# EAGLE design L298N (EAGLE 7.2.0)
CNAME: L298 STEPPER MOTOR BOARD; CREVISION: 1.0; DESIGNER: RODNEYD
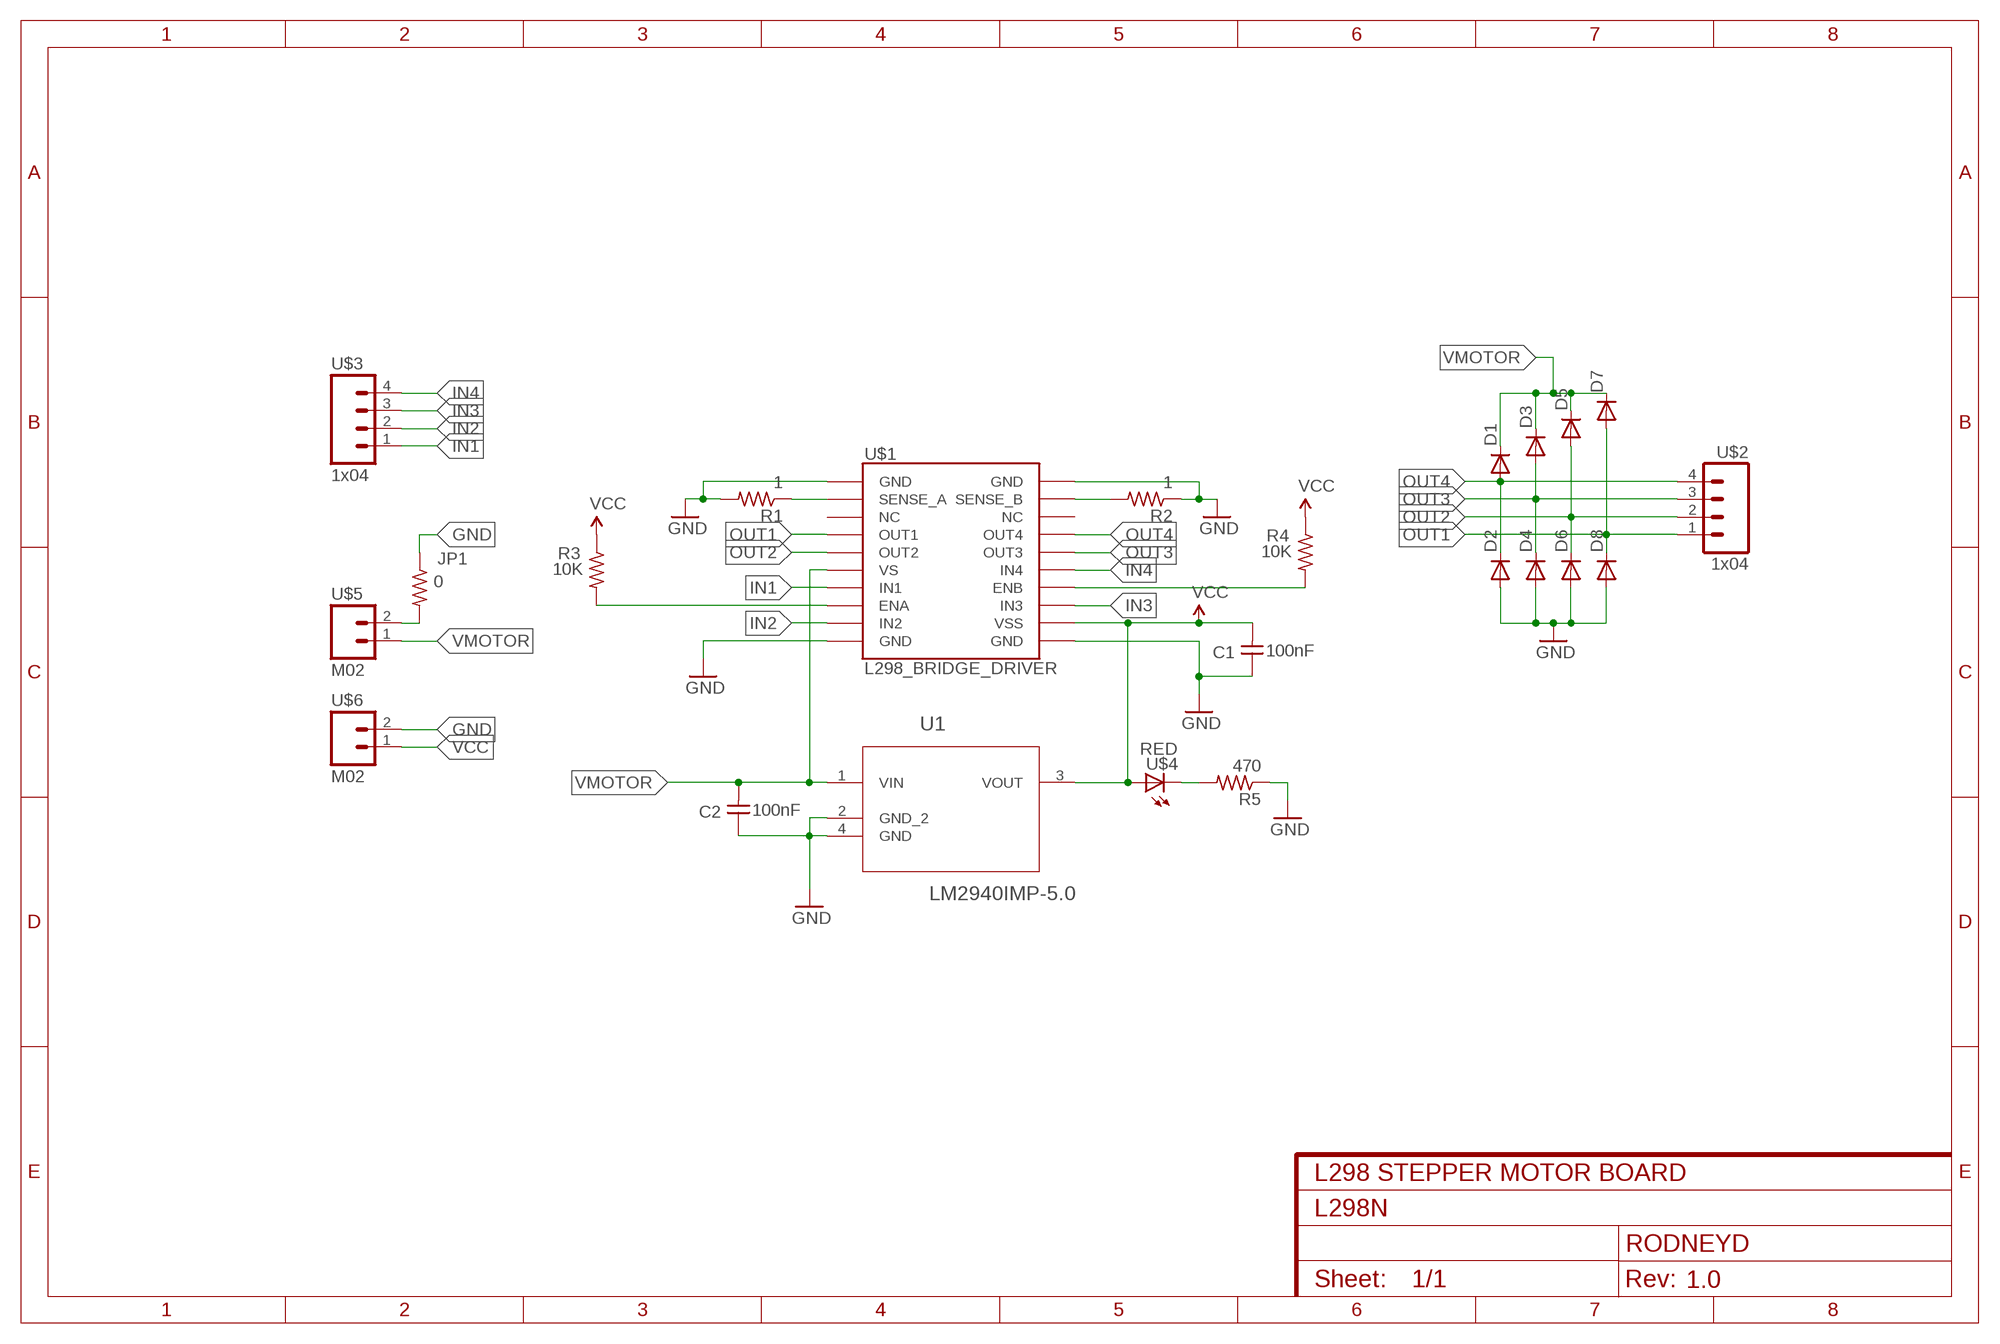
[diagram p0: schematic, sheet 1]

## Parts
C1  100nF  CAPFAB  [C1206FAB]
C2  100nF  CAPFAB  [C1206FAB]
D1  DIODESOD123  [SOD123]
D2  DIODESOD123  [SOD123]
D3  DIODESOD123  [SOD123]
D4  DIODESOD123  [SOD123]
D5  DIODESOD123  [SOD123]
D6  DIODESOD123  [SOD123]
D7  DIODESOD123  [SOD123]
D8  DIODESOD123  [SOD123]
JP1  0  RESISTOR1206FAB  [R1206FAB]
R1  1  RESISTOR1206FAB  [R1206FAB]
R2  1  RESISTOR1206FAB  [R1206FAB]
R3  10K  RESISTOR1206FAB  [R1206FAB]
R4  10K  RESISTOR1206FAB  [R1206FAB]
R5  470  RESISTOR1206FAB  [R1206FAB]
U1  LM2940IMP-5.0  [SOT230P696X180-4N]
U$1  L298_BRIDGE_DRIVER  [POWERSO20]
U$2  1x04  M041X04_SMD_STRAIGHT_ALT  [1X04_SMD_STRAIGHT_ALT]
U$3  1x04  M041X04_SMD_STRAIGHT_ALT  [1X04_SMD_STRAIGHT_ALT]
U$4  RED  LED  [LED1206]
U$5  M02  [1X02_SMD_FLAT_PADS]
U$6  M02  [1X02_SMD_FLAT_PADS]

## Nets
GND: C1.1 C2.1 D2.ANODE(A) D4.ANODE(A) D6.ANODE(A) D8.ANODE(A) JP1.1 R1.2 R2.1 R5.1 U1.2(GND_2) U1.4(GND) U$1.1(GND) U$1.10(GND) U$1.11(GND) U$1.20(GND) U$6.2
IN1: U$1.7(IN1) U$3.1
IN2: U$1.9(IN2) U$3.2
IN3: U$1.13(IN3) U$3.3
IN4: U$1.15(IN4) U$3.4
N$1: R1.1 U$1.2(SENSE_A)
N$2: R2.2 U$1.19(SENSE_B)
N$3: R3.2 U$1.8(ENA)
N$4: R4.2 U$1.14(ENB)
N$5: R5.2 U$4.2(C)
N$6: JP1.2 U$5.2
OUT1: D7.ANODE(A) D8.CATHODE(C) U$1.4(OUT1) U$2.1
OUT2: D5.ANODE(A) D6.CATHODE(C) U$1.5(OUT2) U$2.2
OUT3: D3.ANODE(A) D4.CATHODE(C) U$1.16(OUT3) U$2.3
OUT4: D1.ANODE(A) D2.CATHODE(C) U$1.17(OUT4) U$2.4
VCC: C1.2 R3.1 R4.1 U1.3(VOUT) U$1.12(VSS) U$4.1(A) U$6.1
VMOTOR: C2.2 D1.CATHODE(C) D3.CATHODE(C) D5.CATHODE(C) D7.CATHODE(C) U1.1(VIN) U$1.6(VS) U$5.1
Unconnected: U$1.3(NC) U$1.18(NC)

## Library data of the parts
C1 C2 = Working:CAP
D1-D8 = Working:DIODE: DIODE
JP1 R1-R5 = Working:RESISTOR: Resistor (US Symbol)
U1 = Working:LM2940IMP-5.0: Low Dropout Regulator; MPN: LM2940IMP-50; OC_FARNELL: 9778845; OC_NEWARK: 41K4582; PACKAGE: SOT-223-4; SUPPLIER: National
U$1 = Working:L298_BRIDGE_DRIVER: Full-bridge power driver IC
U$2 U$3 = Working:M04
U$4 = Working:LED: LED
U$5 U$6 = Working:M02

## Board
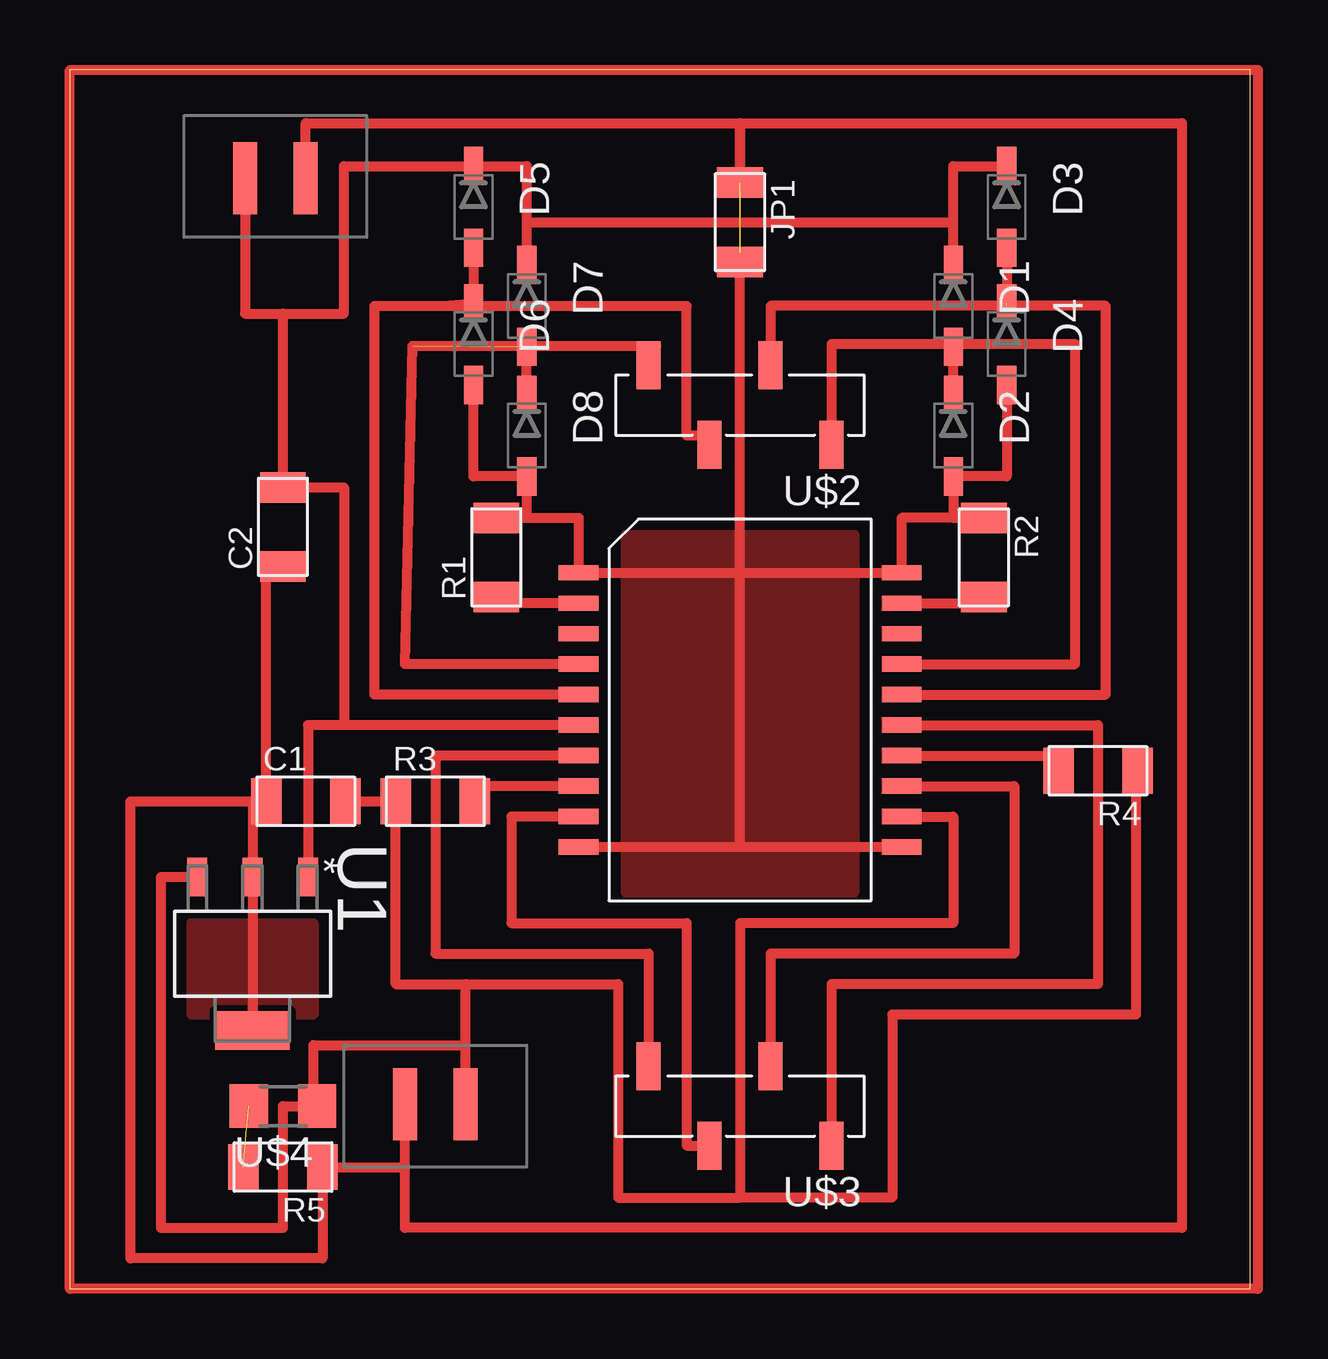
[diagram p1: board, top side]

Size 49.2 x 50.79 mm. Coordinates in mm from the lower left corner, seen from the top.
Outline: 0,0 49.2,0 49.2,50.79 0,50.79 0,0
Copper layers (1*16): Top 0.035mm / dielectric 1.5mm / Bottom 0.035mm
Design rules "default": minimum track width 10mil, minimum drill 24mil, track to track 8mil, track to pad 8mil, pad to pad 8mil, via to via 8mil, smd to smd 8mil, copper to edge 40mil, drill to drill 8mil, minimum pad ring 10mil, minimum via ring 8mil, stop-mask expansion 4mil, vias tented up to drill 0mil, thermal gap 10mil

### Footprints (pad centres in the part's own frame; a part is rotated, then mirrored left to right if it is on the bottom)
C1206FAB = smd 1.27 x 1.905: 1 -1.651,0; 2 1.651,0
SOD123 = smd 1.6 x 0.8: ANODE 1.7,0; CATHODE -1.7,0
R1206FAB = smd 1.27 x 1.905: 1 -1.651,0; 2 1.651,0
SOT230P696X180-4N = smd 1.6 x 0.838: 1 -3.2,2.311; 2 -3.2,0; 3 -3.2,-2.311 | smd 1.6 x 3.099: 4 3.2,0
POWERSO20 = smd 1.651 x 0.635: 1 -6.731,5.715; 2 -6.731,4.445; 3 -6.731,3.175; 4 -6.731,1.905; 5 -6.731,0.635; 6 -6.731,-0.635; 7 -6.731,-1.905; 8 -6.731,-3.175; 9 -6.731,-4.445; 10 -6.731,-5.715; 11 6.731,-5.715; 12 6.731,-4.445; 13 6.731,-3.175; 14 6.731,-1.905; 15 6.731,-0.635; 16 6.731,0.635; 17 6.731,1.905; 18 6.731,3.175; 19 6.731,4.445; 20 6.731,5.715
1X04_SMD_STRAIGHT_ALT = smd 1 x 2: 1 -1.27,-0.38; 2 -3.81,2.92; 3 -6.35,-0.38; 4 -8.89,2.92
LED1206 = smd 1.6 x 1.803: 1 -1.422,0; 2 1.422,0
1X02_SMD_FLAT_PADS = smd 1 x 3: 1 2.54,1.19; 2 5.08,1.19

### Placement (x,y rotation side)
C1  9.84,20.32 0 top
C2  8.89,31.75 90 top
D1  36.83,40.96 270 top
D2  36.83,35.56 270 top
D3  39.05,45.09 270 top
D4  39.05,39.37 270 top
D5  16.83,45.09 270 top
D6  16.83,39.37 270 top
D7  19.05,40.96 270 top
D8  19.05,35.56 270 top
JP1  27.94,44.45 270 top
R1  17.78,30.48 90 top
R2  38.1,30.48 270 top
R3  15.24,20.32 0 top
R4  42.86,21.59 180 top
R5  8.89,5.08 180 top
U1  7.62,13.97 270 top
U$1  27.94,24.13 0 top
U$2  22.86,38.1 180 top
U$3  22.86,8.89 180 top
U$4  8.89,7.62 180 top
U$5  4.76,45.09 0 top
U$6  19.05,8.89 180 top

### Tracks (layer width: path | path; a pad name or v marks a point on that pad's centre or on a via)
GND  (1 unrouted)
  Top 0.406: 27.94,29.84 U$1.1 21.21,32.13 19.05,32.13 | 27.94,29.84 U$1.20 34.67,32.13 R2.1 36.83,32.13 D2.ANODE 39.05,33.86 D4.ANODE | 27.94,18.41 U$1.11 | 27.94,18.41 27.94,29.84 | R1.2 19.05,32.13 | 19.05,32.13 D8.ANODE 16.83,33.86 D6.ANODE | U$1.10 27.94,18.41 | 27.94,29.84 27.94,43.18 | JP1.1 27.94,48.58 46.35,48.58 46.35,2.54 13.97,2.54 13.97,5.08 | U1.4 U1.2 7.62,20.32 | 7.62,20.32 C1.1 8.19,30.1 C2.1 | 13.97,5.08 U$6.2 | 13.97,5.08 R5.1 10.54,1.27 2.54,1.27 2.54,20.32 7.62,20.32
  pour Top: 23.18,31.43 32.7,31.43 32.7,16.51 23.18,16.51
  pour Top: 5.08,15.24 10.16,15.24 10.16,11.43 5.08,11.43
IN1
  Top 0.406: U$1.7 15.24,22.23 15.24,13.97 24.13,13.97 U$3.1
IN2
  Top 0.406: U$1.9 18.41,19.68 18.41,15.24 25.72,15.24 25.72,5.97 U$3.2
IN3
  Top 0.406: U$1.13 39.37,20.95 39.37,13.97 29.21,13.97 U$3.3
IN4
  Top 0.406: U$1.15 42.86,23.5 42.86,12.7 31.75,12.7 U$3.4
N$1
  Top 0.406: U$1.2 17.78,28.57 R1.1
N$2
  Top 0.406: U$1.19 38.1,28.57 R2.2
N$3
  Top 0.406: U$1.8 16.89,20.95 R3.2
N$4
  Top 0.406: U$1.14 41.21,22.23 R4.2
N$5  (1 unrouted)
N$6  (1 unrouted)
  Top 0.406: JP1.2 27.94,43.18 | U$5.2 9.84,48.58 27.94,48.58 27.94,45.72
N$7
  Top 0.406: 0,0 0,50.8 49.53,50.8 49.53,0 0,0
OUT1  (1 unrouted)
  Top 0.406: U$1.4 13.97,26.04 14.29,39.29 24.45,39.29 U$2.1 | D8.CATHODE D7.ANODE
OUT2
  Top 0.406: U$1.5 12.7,24.77 12.7,40.96 15.56,40.96 | 15.56,40.96 25.72,40.96 25.72,35.56 26.67,35.56 U$2.2 | D5.ANODE D6.CATHODE 15.56,40.96
OUT3  (1 unrouted)
  Top 0.406: U$1.16 43.18,24.77 43.18,40.96 39.05,40.96 | 39.05,40.96 29.21,40.96 U$2.3 | D3.ANODE 39.05,40.96
OUT4
  Top 0.406: U$1.17 41.91,26.04 41.91,39.37 36.83,39.37 | 36.83,39.37 31.75,39.37 U$2.4 | 36.83,39.37 D1.ANODE D2.CATHODE
VCC
  Top 0.406: U$1.12 36.83,19.68 36.83,15.24 27.94,15.24 27.94,3.81 | 27.94,3.81 22.86,3.81 22.86,12.7 16.51,12.7 | 44.45,22.23 R4.1 44.45,21.59 44.45,11.43 34.29,11.43 34.29,3.81 27.94,3.81 | U1.3 3.81,17.17 3.81,2.54 8.89,2.54 8.89,7.62 U$4.1 10.16,7.62 10.16,10.16 16.51,10.16 | 16.51,12.7 13.59,12.7 R3.1 C1.2 11.43,20.32 | U$6.1 16.51,10.16 | 16.51,10.16 16.51,12.7
VMOTOR
  Top 0.406: D1.CATHODE 36.83,44.45 | 36.83,44.45 36.83,46.78 D3.CATHODE | 19.05,44.45 19.05,46.78 D5.CATHODE 11.43,46.78 11.43,40.64 8.89,40.64 | 19.05,44.45 D7.CATHODE | 19.05,44.45 36.83,44.45 | U$5.1 7.3,40.64 8.89,40.64 | 8.89,40.64 C2.2 11.43,33.4 11.43,23.5 | U$1.6 11.43,23.5 | 11.43,23.5 9.93,23.5 U1.1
